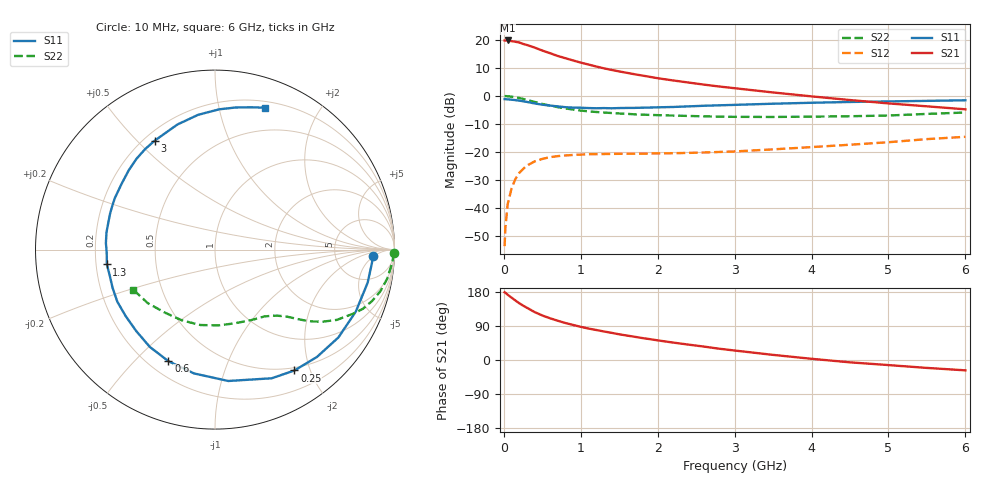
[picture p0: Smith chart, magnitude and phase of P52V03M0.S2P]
! SIEMENS Small Signal Semiconductors
! BFP183
! Si NPN RF Bipolar Junction Transistor in SOT143
! VCE = 2 V  IC = 3 mA
! Common Emitter S-Parameters:  March  1996
# GHz  S  MA  R  50
!  f  S11  S21  S12  S22
! GHz  MAG  ANG  MAG  ANG  MAG  ANG  MAG  ANG
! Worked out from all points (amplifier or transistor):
!   36 points, 10 MHz to 6 GHz, reference 50 ohm
!   highest |S21| = 19.8 dB at 50 MHz (marker M1)
!   |S21| within 3 dB of that: start of sweep to 443.8 MHz
!   unconditionally stable (mu >= 1): 1.841 GHz to 5.768 GHz
!   at 250 MHz: K = 0.15, MSG = 22.3 dB, |S12| = -26.0 dB
!   at 1.4 GHz: K = 0.80, MSG = 15.0 dB, |S12| = -20.7 dB
!   at 6 GHz: K = 0.96, MSG = 4.9 dB, |S12| = -14.6 dB
!   lowest NFmin = 1.10 dB at 450 MHz
!   S11 on the Smith chart (normalised r, x): 10 MHz: 14, -5; 250 MHz: 0.46, -1.76; 600 MHz: 0.28, -0.63; 1.3 GHz: 0.24, -0.06; 3 GHz: 0.24, +0.56; 6 GHz: 0.26, +1.38
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0.01  0.88 -2.4  9.744 178.7  0.0021 88.3  0.9968 -1.0
0.02  0.8778 -4.8  9.749 177.4  0.0045 82.6  0.9955 -2.0
0.05  0.8703 -12.2  9.768 172.2  0.0118 86.2  0.988 -4.8
0.15  0.8441 -35.4  9.257 157.1  0.033 71.2  0.9506 -14.1
0.2  0.8248 -46.5  8.992 149.9  0.0425 65.2  0.9202 -18.2
0.25  0.8058 -56.7  8.476 143.5  0.05 60.4  0.8877 -21.8
0.3  0.7835 -66.2  8.108 137.9  0.0574 55.5  0.8514 -24.7
0.4  0.7358 -84.2  7.295 126.5  0.068 47.5  0.7834 -30.0
0.5  0.6998 -99.6  6.457 117.5  0.0755 40.9  0.7219 -33.8
0.6  0.6736 -112.7  5.793 110.1  0.0811 36.1  0.6729 -36.5
0.7  0.6526 -123.8  5.169 103.6  0.0847 32.1  0.6325 -38.5
0.8  0.6312 -134.1  4.716 97.6  0.087 29.2  0.6002 -40.1
1  0.6168 -151.9  3.93 87.5  0.0901 24.5  0.5492 -42.9
1.1  0.6091 -159.6  3.637 83.0  0.0915 23.0  0.5311 -44.1
1.3  0.6082 -172.2  3.113 75.3  0.0922 20.4  0.5066 -46.6
1.7  0.6131 165.9  2.439 61.3  0.0935 18.8  0.471 -52.0
2.2  0.6365 144.9  1.892 46.0  0.0954 19.0  0.4476 -59.7
3  0.694 118.9  1.375 25.0  0.1026 22.0  0.4246 -75.7
3.5  0.7278 106.7  1.155 13.5  0.1117 24.0  0.4226 -87.3
4.5  0.7819 88.3  0.846 -6.2  0.1352 24.5  0.4353 -115.1
5.5  0.8176 75.9  0.654 -20.9  0.1702 21.9  0.479 -141.5
6  0.8382 70.6  0.578 -27.3  0.1871 18.3  0.5073 -153.9
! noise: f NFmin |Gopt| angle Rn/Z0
0.45  1.1  0.37  35  0.3
0.9  1.15  0.34  85  0.23
1.8  1.9  0.35  160  0.13
